| TEXAS INSTRUMENTS INCORPORATED
| Standard Linear and Logic Group
| IBIS Model of SN74SSTU32864
| 25-BIT CONFIGURABLE REGISTERED BUFFER WITH SSTL_18 INPUTS AND OUTPUTS
| This file contains package information for the following:
|  U*BGA 96-pin (GKE) package as [Component] SSTU32864_GKE_11 for the 1:1 Reg
|  U*BGA 96-pin (GKE) package as [Component] SSTU32864_GKE_12A for the 1:2 RegA
|  U*BGA 96-pin (GKE) package as [Component] SSTU32864_GKE_12B for the 1:2 RegB
| This device can be powered at the following Vccs:
|  1.8 volt Vcc
| This file provides unique models under the [Model Selector] for each Vcc.
| For operation at a specific Vcc, select the appropriate model after each
| [Model Selector] keyword.
[IBIS Ver]   3.2
[Comment char]  |_char
[File Name]   sn74sstu32864.ibs
[File Rev]   1.4 | x_die
[Date]   September 24, 2002
[Source]   Data created from TI-SPICE simulations at TI-SLL.
[Notes]   The following is an IBIS list for the SSTU32864.
   Please contact sllibis@ti.com with questions and
   comments concerning SLL IBIS models.
   An IBIS model does not adequately simulate the dynamic
   behavior of the multi-stage output driver in the SN74SSTU32864
   device. TI recommends that customers do NOT use the IBIS model.
   For more accurate simulation results, please use the HSPICE
   model if you can.
[Disclaimer] Property of Texas Instruments Incorporated.  Unauthorized
   reproduction and/or distribution is strictly prohibited.
   This product is protected under copyright law.
   Created  2002, (C) Copyright  2002, Texas Instruments
   Incorporated, All Rights Reserved
   UNLESS THERE IS A SIGNED, WRITTEN AGREEMENT TO THE
   CONTRARY, TEXAS INSTRUMENTS (TI) IS PROVIDING THE IBIS
   MODELS  AND WITHOUT ANY WARRANTY, EXPRESSED OR
   IMPLIED.  TI assumes no liability for:
   1) the accuracy of the IBIS models provided to your
   company;
   2) the proper functioning of these IBIS Models in your
   design or for any resulting applications; or
   3) infringement of patents, copyrights or intellectual
   property rights resulting from your use of these IBIS
   models.
   TI provides IBIS Models as a service to our customers.
   You and your company shall not distribute, sell or give
   these models to anyone else without prior written
   permission from TI.
   TI reserves the right to make changes to our products or
   to discontinue any semiconductor product or service
   without notice, and advises our customers to obtain the
   latest version of relevant information to verify, before
   placing orders, that the information being relied on is
   current.
   Please be aware that your receipt and use of the IBIS
   information provided shall serve as acceptance of these
   terms and conditions.  If you do not accept these terms,
   you should return or destroy the IBIS models and any
   other accompanying information immediately.
| Component SSTU32864_GKE_11 96-pin U*BGA
[Component]   SSTU32864_GKE_11
[Manufacturer]   Texas Instruments, Inc.
[Package]
|   typ   min   max
R_pkg   5.800e-02   4.400e-02   8.900e-02
L_pkg   2.237e-09   1.365e-09   3.243e-09
C_pkg   2.190e-13   1.460e-13   3.240e-13
[Pin]   signal_name   model_name   R_pin   L_pin   C_pin
A3   VREF   SSTU32864_VREF   8.200e-02   2.543e-09   1.960e-13
B3   GND   GND   6.600e-02   1.828e-09   1.670e-13
A2   DNU   NC   8.900e-02   2.721e-09   1.970e-13
A1   DCKE   SSTU32864_DCKE   4.900e-02   2.740e-09   2.590e-13
B2   D15   SSTU32864_D   5.200e-02   2.647e-09   2.840e-13
B1   D2   SSTU32864_D   5.000e-02   2.563e-09   3.000e-13
C3   VCC   POWER   6.200e-02   2.921e-09   3.240e-13
C2   D16   SSTU32864_D   5.300e-02   2.399e-09   2.730e-13
C1   D3   SSTU32864_D   5.000e-02   2.223e-09   2.350e-13
D3   GND   GND   6.800e-02   2.959e-09   2.840e-13
D2   DNU   NC   5.100e-02   2.149e-09   2.250e-13
D1   DODT   SSTU32864_DODT   4.900e-02   2.019e-09   2.080e-13
E3   VCC   POWER   7.000e-02   2.832e-09   2.660e-13
E2   D17   SSTU32864_D   5.100e-02   1.969e-09   2.020e-13
E1   D5   SSTU32864_D   5.100e-02   1.876e-09   1.880e-13
F3   GND   GND   6.700e-02   2.521e-09   2.300e-13
F2   D18   SSTU32864_D   4.700e-02   1.609e-09   1.640e-13
F1   D6   SSTU32864_D   4.900e-02   1.661e-09   1.690e-13
G3   VCC   POWER   6.800e-02   2.403e-09   2.200e-13
G2   NRESET   SSTU32864_RESET   4.800e-02   1.559e-09   1.580e-13
G1   NC   NC   5.100e-02   1.567e-09   1.610e-13
H3   GND   GND   6.600e-02   2.241e-09   2.020e-13
H2   DCS   SSTU32864_DCS   5.000e-02   1.530e-09   1.490e-13
H1   CLK   SSTU32864_CLK   5.100e-02   1.581e-09   1.510e-13
J1   NCLK   SSTU32864_CLK   5.100e-02   1.589e-09   1.600e-13
J2   CSR   SSTU32864_DCS   4.400e-02   1.365e-09   1.460e-13
J3   VCC   POWER   6.600e-02   2.240e-09   2.060e-13
K1   D8   SSTU32864_D   5.000e-02   1.565e-09   1.620e-13
K2   D19   SSTU32864_D   4.900e-02   1.560e-09   1.580e-13
K3   GND   GND   6.900e-02   2.405e-09   2.200e-13
L1   D9   SSTU32864_D   5.000e-02   1.663e-09   1.690e-13
L2   D20   SSTU32864_D   4.800e-02   1.610e-09   1.630e-13
L3   VCC   POWER   6.700e-02   2.522e-09   2.300e-13
M1   D10   SSTU32864_D   5.100e-02   1.876e-09   1.880e-13
M2   D21   SSTU32864_D   5.100e-02   1.969e-09   2.020e-13
M3   GND   GND   6.900e-02   2.831e-09   2.660e-13
N1   D11   SSTU32864_D   5.000e-02   2.019e-09   2.080e-13
N2   D22   SSTU32864_D   5.100e-02   2.149e-09   2.250e-13
N3   VCC   POWER   6.800e-02   2.959e-09   2.840e-13
P1   D12   SSTU32864_D   5.000e-02   2.223e-09   2.350e-13
P2   D23   SSTU32864_D   5.300e-02   2.400e-09   2.700e-13
P3   GND   GND   6.200e-02   2.916e-09   3.230e-13
R1   D13   SSTU32864_D   5.000e-02   2.560e-09   3.030e-13
R2   D24   SSTU32864_D   5.200e-02   2.644e-09   2.860e-13
T1   D14   SSTU32864_D   4.900e-02   2.729e-09   2.880e-13
T2   D25   SSTU32864_D   5.800e-02   3.113e-09   2.710e-13
R3   VCC   POWER   7.500e-02   2.106e-09   1.560e-13
T3   VREF   SSTU32864_VREF   8.200e-02   2.543e-09   1.960e-13
T4   VCC   POWER   8.200e-02   2.541e-09   2.100e-13
R4   VCC   POWER   6.600e-02   1.828e-09   1.670e-13
T5   Q14   SSTU32864_Q   8.900e-02   2.722e-09   1.920e-13
T6   Q25   SSTU32864_Q   4.900e-02   2.735e-09   2.570e-13
R5   Q13   SSTU32864_Q   5.200e-02   2.643e-09   2.800e-13
R6   Q24   SSTU32864_Q   5.000e-02   2.567e-09   2.740e-13
P4   GND   GND   6.800e-02   3.243e-09   3.120e-13
P5   Q12   SSTU32864_Q   5.300e-02   2.495e-09   2.580e-13
P6   Q23   SSTU32864_Q   5.000e-02   2.303e-09   2.470e-13
N4   VCC   POWER   6.800e-02   3.020e-09   2.930e-13
N5   Q11   SSTU32864_Q   5.100e-02   2.212e-09   2.300e-13
N6   Q22   SSTU32864_Q   4.900e-02   2.081e-09   2.130e-13
M4   GND   GND   7.000e-02   2.893e-09   2.710e-13
M5   Q10   SSTU32864_Q   5.100e-02   2.028e-09   2.070e-13
M6   Q21   SSTU32864_Q   5.100e-02   1.932e-09   1.950e-13
L4   VCC   POWER   6.700e-02   2.558e-09   2.320e-13
L5   Q9   SSTU32864_Q   4.700e-02   1.659e-09   1.690e-13
L6   Q20   SSTU32864_Q   4.900e-02   1.676e-09   1.730e-13
K4   GND   GND   6.800e-02   2.418e-09   2.200e-13
K5   Q8   SSTU32864_Q   4.900e-02   1.572e-09   1.580e-13
K6   Q19   SSTU32864_Q   5.000e-02   1.577e-09   1.610e-13
J4   VCC   POWER   6.600e-02   2.253e-09   2.010e-13
J5   NC   NC   5.000e-02   1.533e-09   1.490e-13
J6   NC   NC   5.100e-02   1.580e-09   1.580e-13
H6   NC   NC   5.100e-02   1.580e-09   1.580e-13
H5   QCS   SSTU32864_QCS   5.000e-02   1.531e-09   1.490e-13
H4   GND   GND   6.600e-02   2.251e-09   2.010e-13
G6   C0   SSTU32864_CNT   5.000e-02   1.576e-09   1.610e-13
G5   C1   SSTU32864_CNT   4.900e-02   1.572e-09   1.580e-13
G4   VCC   POWER   6.800e-02   2.418e-09   2.200e-13
F6   Q18   SSTU32864_Q   4.900e-02   1.676e-09   1.730e-13
F5   Q6   SSTU32864_Q   4.700e-02   1.659e-09   1.690e-13
F4   GND   GND   6.700e-02   2.557e-09   2.320e-13
E6   Q17   SSTU32864_Q   5.100e-02   1.932e-09   1.950e-13
E5   Q5   SSTU32864_Q   5.100e-02   2.029e-09   2.070e-13
E4   VCC   POWER   6.900e-02   2.892e-09   2.710e-13
D6   DNU   NC   5.000e-02   2.082e-09   2.130e-13
D5   QODT   SSTU32864_QODT   5.100e-02   2.212e-09   2.300e-13
D4   GND   GND   6.800e-02   3.021e-09   2.930e-13
C6   Q16   SSTU32864_Q   5.000e-02   2.304e-09   2.460e-13
C5   Q3   SSTU32864_Q   5.300e-02   2.495e-09   2.580e-13
C4   VCC   POWER   6.900e-02   3.243e-09   3.120e-13
B6   Q15   SSTU32864_Q   5.000e-02   2.566e-09   2.740e-13
B5   Q2   SSTU32864_Q   5.200e-02   2.642e-09   2.800e-13
A6   DNU   NC   4.900e-02   2.735e-09   2.570e-13
A5   QCKE   SSTU32864_QCKE   8.900e-02   2.722e-09   1.950e-13
B4   GND   GND   6.600e-02   1.828e-09   1.690e-13
A4   VCC   POWER   8.200e-02   2.542e-09   2.000e-13
| Component SSTU32864_GKE_12A 96-pin U*BGA
[Component]   SSTU32864_GKE_12A
[Manufacturer]   Texas Instruments, Inc.
[Package]
|   typ   min   max
R_pkg   5.800e-02   4.400e-02   8.900e-02
L_pkg   2.237e-09   1.365e-09   3.243e-09
C_pkg   2.190e-13   1.460e-13   3.240e-13
[Pin]   signal_name   model_name   R_pin   L_pin   C_pin
A3   VREF   SSTU32864_VREF   8.200e-02   2.543e-09   1.960e-13
B3   GND   GND   6.600e-02   1.828e-09   1.670e-13
A2   DNU   NC   8.900e-02   2.721e-09   1.970e-13
A1   DCKE   SSTU32864_DCKE   4.900e-02   2.740e-09   2.590e-13
B2   DNU   NC   5.200e-02   2.647e-09   2.840e-13
B1   D2   SSTU32864_D   5.000e-02   2.563e-09   3.000e-13
C3   VCC   POWER   6.200e-02   2.921e-09   3.240e-13
C2   DNU   NC   5.300e-02   2.399e-09   2.730e-13
C1   D3   SSTU32864_D   5.000e-02   2.223e-09   2.350e-13
D3   GND   GND   6.800e-02   2.959e-09   2.840e-13
D2   DNU   NC   5.100e-02   2.149e-09   2.250e-13
D1   DODT   SSTU32864_DODT   4.900e-02   2.019e-09   2.080e-13
E3   VCC   POWER   7.000e-02   2.832e-09   2.660e-13
E2   DNU   NC   5.100e-02   1.969e-09   2.020e-13
E1   D5   SSTU32864_D   5.100e-02   1.876e-09   1.880e-13
F3   GND   GND   6.700e-02   2.521e-09   2.300e-13
F2   DNU   NC   4.700e-02   1.609e-09   1.640e-13
F1   D6   SSTU32864_D   4.900e-02   1.661e-09   1.690e-13
G3   VCC   POWER   6.800e-02   2.403e-09   2.200e-13
G2   NRESET   SSTU32864_RESET   4.800e-02   1.559e-09   1.580e-13
G1   NC   NC   5.100e-02   1.567e-09   1.610e-13
H3   GND   GND   6.600e-02   2.241e-09   2.020e-13
H2   DCS   SSTU32864_DCS   5.000e-02   1.530e-09   1.490e-13
H1   CLK   SSTU32864_CLK   5.100e-02   1.581e-09   1.510e-13
J1   NCLK   SSTU32864_CLK   5.100e-02   1.589e-09   1.600e-13
J2   CSR   SSTU32864_DCS   4.400e-02   1.365e-09   1.460e-13
J3   VCC   POWER   6.600e-02   2.240e-09   2.060e-13
K1   D8   SSTU32864_D   5.000e-02   1.565e-09   1.620e-13
K2   DNU   NC   4.900e-02   1.560e-09   1.580e-13
K3   GND   GND   6.900e-02   2.405e-09   2.200e-13
L1   D9   SSTU32864_D   5.000e-02   1.663e-09   1.690e-13
L2   DNU   NC   4.800e-02   1.610e-09   1.630e-13
L3   VCC   POWER   6.700e-02   2.522e-09   2.300e-13
M1   D10   SSTU32864_D   5.100e-02   1.876e-09   1.880e-13
M2   DNU   NC   5.100e-02   1.969e-09   2.020e-13
M3   GND   GND   6.900e-02   2.831e-09   2.660e-13
N1   D11   SSTU32864_D   5.000e-02   2.019e-09   2.080e-13
N2   DNU   NC   5.100e-02   2.149e-09   2.250e-13
N3   VCC   POWER   6.800e-02   2.959e-09   2.840e-13
P1   D12   SSTU32864_D   5.000e-02   2.223e-09   2.350e-13
P2   DNU   NC   5.300e-02   2.400e-09   2.700e-13
P3   GND   GND   6.200e-02   2.916e-09   3.230e-13
R1   D13   SSTU32864_D   5.000e-02   2.560e-09   3.030e-13
R2   DNU   NC   5.200e-02   2.644e-09   2.860e-13
T1   D14   SSTU32864_D   4.900e-02   2.729e-09   2.880e-13
T2   DNU   NC   5.800e-02   3.113e-09   2.710e-13
R3   VCC   POWER   7.500e-02   2.106e-09   1.560e-13
T3   VREF   SSTU32864_VREF   8.200e-02   2.543e-09   1.960e-13
T4   VCC   POWER   8.200e-02   2.541e-09   2.100e-13
R4   VCC   POWER   6.600e-02   1.828e-09   1.670e-13
T5   Q14A   SSTU32864_Q   8.900e-02   2.722e-09   1.920e-13
T6   Q14B   SSTU32864_Q   4.900e-02   2.735e-09   2.570e-13
R5   Q13A   SSTU32864_Q   5.200e-02   2.643e-09   2.800e-13
R6   Q13B   SSTU32864_Q   5.000e-02   2.567e-09   2.740e-13
P4   GND   GND   6.800e-02   3.243e-09   3.120e-13
P5   Q12A   SSTU32864_Q   5.300e-02   2.495e-09   2.580e-13
P6   Q12B   SSTU32864_Q   5.000e-02   2.303e-09   2.470e-13
N4   VCC   POWER   6.800e-02   3.020e-09   2.930e-13
N5   Q11A   SSTU32864_Q   5.100e-02   2.212e-09   2.300e-13
N6   Q11B   SSTU32864_Q   4.900e-02   2.081e-09   2.130e-13
M4   GND   GND   7.000e-02   2.893e-09   2.710e-13
M5   Q10A   SSTU32864_Q   5.100e-02   2.028e-09   2.070e-13
M6   Q10B   SSTU32864_Q   5.100e-02   1.932e-09   1.950e-13
L4   VCC   POWER   6.700e-02   2.558e-09   2.320e-13
L5   Q9A   SSTU32864_Q   4.700e-02   1.659e-09   1.690e-13
L6   Q9B   SSTU32864_Q   4.900e-02   1.676e-09   1.730e-13
K4   GND   GND   6.800e-02   2.418e-09   2.200e-13
K5   Q8A   SSTU32864_Q   4.900e-02   1.572e-09   1.580e-13
K6   Q8B   SSTU32864_Q   5.000e-02   1.577e-09   1.610e-13
J4   VCC   POWER   6.600e-02   2.253e-09   2.010e-13
J5   NC   NC   5.000e-02   1.533e-09   1.490e-13
J6   NC   NC   5.100e-02   1.580e-09   1.580e-13
H6   QCSB   SSTU32864_QCS   5.100e-02   1.580e-09   1.580e-13
H5   QCSA   SSTU32864_QCS   5.000e-02   1.531e-09   1.490e-13
H4   GND   GND   6.600e-02   2.251e-09   2.010e-13
G6   C0   SSTU32864_CNT   5.000e-02   1.576e-09   1.610e-13
G5   C1   SSTU32864_CNT   4.900e-02   1.572e-09   1.580e-13
G4   VCC   POWER   6.800e-02   2.418e-09   2.200e-13
F6   Q6B   SSTU32864_Q   4.900e-02   1.676e-09   1.730e-13
F5   Q6A   SSTU32864_Q   4.700e-02   1.659e-09   1.690e-13
F4   GND   GND   6.700e-02   2.557e-09   2.320e-13
E6   Q5B   SSTU32864_Q   5.100e-02   1.932e-09   1.950e-13
E5   Q5A   SSTU32864_Q   5.100e-02   2.029e-09   2.070e-13
E4   VCC   POWER   6.900e-02   2.892e-09   2.710e-13
D6   QODTB   SSTU32864_QODT   5.000e-02   2.082e-09   2.130e-13
D5   QODTA   SSTU32864_QODT   5.100e-02   2.212e-09   2.300e-13
D4   GND   GND   6.800e-02   3.021e-09   2.930e-13
C6   Q3B   SSTU32864_Q   5.000e-02   2.304e-09   2.460e-13
C5   Q3A   SSTU32864_Q   5.300e-02   2.495e-09   2.580e-13
C4   VCC   POWER   6.900e-02   3.243e-09   3.120e-13
B6   Q2B   SSTU32864_Q   5.000e-02   2.566e-09   2.740e-13
B5   Q2A   SSTU32864_Q   5.200e-02   2.642e-09   2.800e-13
A6   QCKEB   SSTU32864_QCKE   4.900e-02   2.735e-09   2.570e-13
A5   QCKEA   SSTU32864_QCKE   8.900e-02   2.722e-09   1.950e-13
B4   GND   GND   6.600e-02   1.828e-09   1.690e-13
A4   VCC   POWER   8.200e-02   2.542e-09   2.000e-13
| Component SSTU32864_GKE_12B 96-pin U*BGA
[Component]   SSTU32864_GKE_12B
[Manufacturer]   Texas Instruments, Inc.
[Package]
|   typ   min   max
R_pkg   5.800e-02   4.400e-02   8.900e-02
L_pkg   2.237e-09   1.365e-09   3.243e-09
C_pkg   2.190e-13   1.460e-13   3.240e-13
[Pin]   signal_name   model_name   R_pin   L_pin   C_pin
A3   VREF   SSTU32864_VREF   8.200e-02   2.543e-09   1.960e-13
B3   GND   GND   6.600e-02   1.828e-09   1.670e-13
A2   DNU   NC   8.900e-02   2.721e-09   1.970e-13
A1   D1   SSTU32864_D   4.900e-02   2.740e-09   2.590e-13
B2   DNU   NC   5.200e-02   2.647e-09   2.840e-13
B1   D2   SSTU32864_D   5.000e-02   2.563e-09   3.000e-13
C3   VCC   POWER   6.200e-02   2.921e-09   3.240e-13
C2   DNU   NC   5.300e-02   2.399e-09   2.730e-13
C1   D3   SSTU32864_D   5.000e-02   2.223e-09   2.350e-13
D3   GND   GND   6.800e-02   2.959e-09   2.840e-13
D2   DNU   NC   5.100e-02   2.149e-09   2.250e-13
D1   D4   SSTU32864_D   4.900e-02   2.019e-09   2.080e-13
E3   VCC   POWER   7.000e-02   2.832e-09   2.660e-13
E2   DNU   NC   5.100e-02   1.969e-09   2.020e-13
E1   D5   SSTU32864_D   5.100e-02   1.876e-09   1.880e-13
F3   GND   GND   6.700e-02   2.521e-09   2.300e-13
F2   DNU   NC   4.700e-02   1.609e-09   1.640e-13
F1   D6   SSTU32864_D   4.900e-02   1.661e-09   1.690e-13
G3   VCC   POWER   6.800e-02   2.403e-09   2.200e-13
G2   NRESET   SSTU32864_RESET   4.800e-02   1.559e-09   1.580e-13
G1   NC   NC   5.100e-02   1.567e-09   1.610e-13
H3   GND   GND   6.600e-02   2.241e-09   2.020e-13
H2   DCS   SSTU32864_DCS   5.000e-02   1.530e-09   1.490e-13
H1   CLK   SSTU32864_CLK   5.100e-02   1.581e-09   1.510e-13
J1   NCLK   SSTU32864_CLK   5.100e-02   1.589e-09   1.600e-13
J2   CSR   SSTU32864_DCS   4.400e-02   1.365e-09   1.460e-13
J3   VCC   POWER   6.600e-02   2.240e-09   2.060e-13
K1   D8   SSTU32864_D   5.000e-02   1.565e-09   1.620e-13
K2   DNU   NC   4.900e-02   1.560e-09   1.580e-13
K3   GND   GND   6.900e-02   2.405e-09   2.200e-13
L1   D9   SSTU32864_D   5.000e-02   1.663e-09   1.690e-13
L2   DNU   NC   4.800e-02   1.610e-09   1.630e-13
L3   VCC   POWER   6.700e-02   2.522e-09   2.300e-13
M1   D10   SSTU32864_D   5.100e-02   1.876e-09   1.880e-13
M2   DNU   NC   5.100e-02   1.969e-09   2.020e-13
M3   GND   GND   6.900e-02   2.831e-09   2.660e-13
N1   DODT   SSTU32864_DODT   5.000e-02   2.019e-09   2.080e-13
N2   DNU   NC   5.100e-02   2.149e-09   2.250e-13
N3   VCC   POWER   6.800e-02   2.959e-09   2.840e-13
P1   D12   SSTU32864_D   5.000e-02   2.223e-09   2.350e-13
P2   DNU   NC   5.300e-02   2.400e-09   2.700e-13
P3   GND   GND   6.200e-02   2.916e-09   3.230e-13
R1   D13   SSTU32864_D   5.000e-02   2.560e-09   3.030e-13
R2   DNU   NC   5.200e-02   2.644e-09   2.860e-13
T1   DCKE   SSTU32864_DCKE   4.900e-02   2.729e-09   2.880e-13
T2   DNU   NC   5.800e-02   3.113e-09   2.710e-13
R3   VCC   POWER   7.500e-02   2.106e-09   1.560e-13
T3   VREF   SSTU32864_VREF   8.200e-02   2.543e-09   1.960e-13
T4   VCC   POWER   8.200e-02   2.541e-09   2.100e-13
R4   VCC   POWER   6.600e-02   1.828e-09   1.670e-13
T5   QCKEA   SSTU32864_QCKE   8.900e-02   2.722e-09   1.920e-13
T6   QCKEB   SSTU32864_QCKE   4.900e-02   2.735e-09   2.570e-13
R5   Q13A   SSTU32864_Q   5.200e-02   2.643e-09   2.800e-13
R6   Q13B   SSTU32864_Q   5.000e-02   2.567e-09   2.740e-13
P4   GND   GND   6.800e-02   3.243e-09   3.120e-13
P5   Q12A   SSTU32864_Q   5.300e-02   2.495e-09   2.580e-13
P6   Q12B   SSTU32864_Q   5.000e-02   2.303e-09   2.470e-13
N4   VCC   POWER   6.800e-02   3.020e-09   2.930e-13
N5   QODTA   SSTU32864_QODT   5.100e-02   2.212e-09   2.300e-13
N6   QODTB   SSTU32864_QODT   4.900e-02   2.081e-09   2.130e-13
M4   GND   GND   7.000e-02   2.893e-09   2.710e-13
M5   Q10A   SSTU32864_Q   5.100e-02   2.028e-09   2.070e-13
M6   Q10B   SSTU32864_Q   5.100e-02   1.932e-09   1.950e-13
L4   VCC   POWER   6.700e-02   2.558e-09   2.320e-13
L5   Q9A   SSTU32864_Q   4.700e-02   1.659e-09   1.690e-13
L6   Q9B   SSTU32864_Q   4.900e-02   1.676e-09   1.730e-13
K4   GND   GND   6.800e-02   2.418e-09   2.200e-13
K5   Q8A   SSTU32864_Q   4.900e-02   1.572e-09   1.580e-13
K6   Q8B   SSTU32864_Q   5.000e-02   1.577e-09   1.610e-13
J4   VCC   POWER   6.600e-02   2.253e-09   2.010e-13
J5   NC   NC   5.000e-02   1.533e-09   1.490e-13
J6   NC   NC   5.100e-02   1.580e-09   1.580e-13
H6   QCSB   SSTU32864_QCS   5.100e-02   1.580e-09   1.580e-13
H5   QCSA   SSTU32864_QCS   5.000e-02   1.531e-09   1.490e-13
H4   GND   GND   6.600e-02   2.251e-09   2.010e-13
G6   C0   SSTU32864_CNT   5.000e-02   1.576e-09   1.610e-13
G5   C1   SSTU32864_CNT   4.900e-02   1.572e-09   1.580e-13
G4   VCC   POWER   6.800e-02   2.418e-09   2.200e-13
F6   Q6B   SSTU32864_Q   4.900e-02   1.676e-09   1.730e-13
F5   Q6A   SSTU32864_Q   4.700e-02   1.659e-09   1.690e-13
F4   GND   GND   6.700e-02   2.557e-09   2.320e-13
E6   Q5B   SSTU32864_Q   5.100e-02   1.932e-09   1.950e-13
E5   Q5A   SSTU32864_Q   5.100e-02   2.029e-09   2.070e-13
E4   VCC   POWER   6.900e-02   2.892e-09   2.710e-13
D6   Q4B   SSTU32864_Q   5.000e-02   2.082e-09   2.130e-13
D5   Q4A   SSTU32864_Q   5.100e-02   2.212e-09   2.300e-13
D4   GND   GND   6.800e-02   3.021e-09   2.930e-13
C6   Q3B   SSTU32864_Q   5.000e-02   2.304e-09   2.460e-13
C5   Q3A   SSTU32864_Q   5.300e-02   2.495e-09   2.580e-13
C4   VCC   POWER   6.900e-02   3.243e-09   3.120e-13
B6   Q2B   SSTU32864_Q   5.000e-02   2.566e-09   2.740e-13
B5   Q2A   SSTU32864_Q   5.200e-02   2.642e-09   2.800e-13
A6   Q1B   SSTU32864_Q   4.900e-02   2.735e-09   2.570e-13
A5   Q1A   SSTU32864_Q   8.900e-02   2.722e-09   1.950e-13
B4   GND   GND   6.600e-02   1.828e-09   1.690e-13
A4   VCC   POWER   8.200e-02   2.542e-09   2.000e-13
| Models and submodels in the file (12): SSTU32864_RESET (Input), SSTU32864_DCS (Input), SSTU32864_D (Input), SSTU32864_VREF (Input), SSTU32864_CNT (Input), SSTU32864_DCKE (Input), SSTU32864_CLK (Input), SSTU32864_DODT (Input), SSTU32864_QODT (Output), SSTU32864_QCS (Output), SSTU32864_QCKE (Output), SSTU32864_Q (Output)
